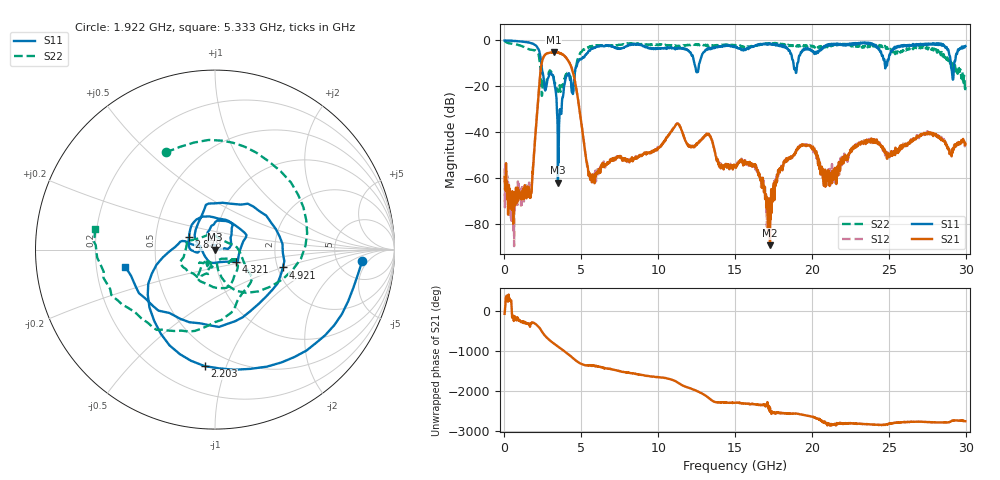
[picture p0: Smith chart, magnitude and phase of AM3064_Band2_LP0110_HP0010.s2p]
# Hz S DB R 50.0
!freq dBS11 angS11 dBS21 angS21 dBS12 angS12 dBS22 angS22
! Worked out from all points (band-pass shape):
!   1600 points, 10 MHz to 29.98 GHz, reference 50 ohm
!   highest |S21| = -5.07 dB at 3.215 GHz (marker M1); lowest = -89.5 dB at 17.27 GHz (marker M2)
!   |S21| within 3 dB of the highest: 2.495 GHz to 4.074 GHz (1.579 GHz wide, 48.1 % of centre)
!   lowest |S11| = -62.1 dB at 3.478 GHz (marker M3), VSWR 1.00, Z = 50 - j0.0729 ohm
!   |S11| at or under -10 dB: 2.399 GHz to 4.738 GHz (2.338 GHz wide, 65.5 % of centre); 12.35 GHz to 12.68 GHz (322.4 MHz wide, 2.58 % of centre); 18.8 GHz to 19.05 GHz (253.3 MHz wide, 1.34 % of centre)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
!   |S22| runs from -24.2 to -0.2 dB; largest |S21 - S12| = 0.018
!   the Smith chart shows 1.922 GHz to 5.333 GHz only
!   S11 on the Smith chart (normalised r, x): 1.922 GHz: 8.83, -3.54; 2.203 GHz: 0.37, -0.84; 2.878 GHz: 0.74, +0.11; 4.321 GHz: 1.25, -0.17; 4.921 GHz: 2.14, -0.50; 5.333 GHz: 0.33, -0.08
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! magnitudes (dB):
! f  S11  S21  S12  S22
! 10 MHz  0.0  -59.8  -56.0  -0.2
! 497.3 MHz  -0.1  -66.2  -68.5  -1.5
! 1.659 GHz  -1.0  -68.8  -66.0  -4.0
! 1.922 GHz  -1.7  -49.3  -49.1  -4.3
! 2.203 GHz  -3.7  -24.5  -24.5  -5.9
! 2.878 GHz  -15.9  -5.5  -5.4  -14.2
! 3.215 GHz  -17.3  -5.1  -5.2  -16.9
! 3.478 GHz  -62.1  -5.2  -5.4  -21.7
! 4.321 GHz  -17.4  -11.2  -11.1  -17.1
! 4.921 GHz  -8.1  -32.1  -32.2  -5.6
! 5.015 GHz  -8.2  -36.7  -36.8  -5.0
! 5.333 GHz  -5.9  -52.8  -52.3  -3.4
! 10 GHz  -3.5  -47.2  -46.8  -1.9
! 11.26 GHz  -3.5  -36.3  -36.3  -2.7
! 15 GHz  -2.7  -55.4  -54.6  -2.1
! 16.34 GHz  -2.3  -54.9  -54.2  -2.3
! 17.27 GHz  -1.5  -89.5  -72.5  -1.4
! 18.25 GHz  -3.2  -52.5  -53.0  -1.8
! 19.99 GHz  -4.4  -46.8  -47.0  -2.3
! 20.85 GHz  -2.7  -56.4  -57.6  -2.8
! 25 GHz  -8.1  -50.7  -49.8  -3.2
! 29.98 GHz  -2.5  -45.1  -45.0  -20.3
